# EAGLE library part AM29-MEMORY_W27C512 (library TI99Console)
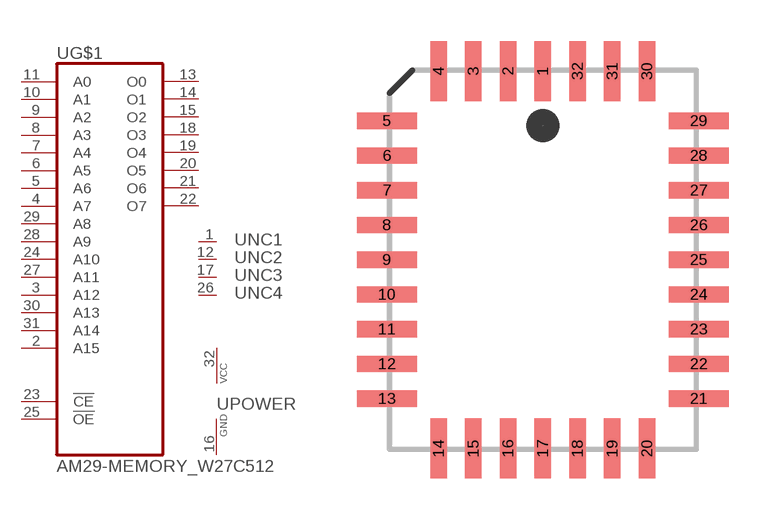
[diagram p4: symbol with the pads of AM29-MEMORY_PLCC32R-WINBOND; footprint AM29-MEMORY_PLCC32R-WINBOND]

Designator prefix -; gates G$1=AM29-MEMORY_W27C512 NC1=NC NC2=NC NC3=NC NC4=NC POWER=VCC-GND

## AM29-MEMORY_W27C512  [AM29-MEMORY_PLCC32R-WINBOND]
1  NC1:NC  nc
2  G$1:A15  in
3  G$1:A12  in
4  G$1:A7  in
5  G$1:A6  in
6  G$1:A5  in
7  G$1:A4  in
8  G$1:A3  in
9  G$1:A2  in
10  G$1:A1  in
11  G$1:A0  in
12  NC2:NC  nc
13  G$1:O0  hiz
14  G$1:O1  hiz
15  G$1:O2  hiz
16  POWER:GND  pwr
17  NC3:NC  nc
18  G$1:O3  hiz
19  G$1:O4  hiz
20  G$1:O5  hiz
21  G$1:O6  hiz
22  G$1:O7  hiz
23  G$1:!CE  in
24  G$1:A10  in
25  G$1:!OE  in
26  NC4:NC  nc
27  G$1:A11  in
28  G$1:A9  in
29  G$1:A8  in
30  G$1:A13  in
31  G$1:A14  in
32  POWER:VCC  pwr

## Footprint AM29-MEMORY_PLCC32R-WINBOND (pad centres in mm)
smd 0.6 x 2.2: 1 0,6.9; 2 -1.27,6.9; 3 -2.54,6.9; 4 -3.81,6.9; 14 -3.81,-6.9; 15 -2.54,-6.9; 16 -1.27,-6.9; 17 0,-6.9; 18 1.27,-6.9; 19 2.54,-6.9; 20 3.81,-6.9; 30 3.81,6.9; 31 2.54,6.9; 32 1.27,6.9
smd 2.2 x 0.6: 5 -5.7,5.08; 6 -5.7,3.81; 7 -5.7,2.54; 8 -5.7,1.27; 9 -5.7,0; 10 -5.7,-1.27; 11 -5.7,-2.54; 12 -5.7,-3.81; 13 -5.7,-5.08; 21 5.7,-5.08; 22 5.7,-3.81; 23 5.7,-2.54; 24 5.7,-1.27; 25 5.7,0; 26 5.7,1.27; 27 5.7,2.54; 28 5.7,3.81; 29 5.7,5.08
